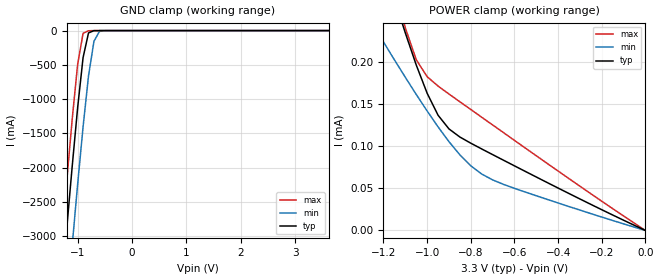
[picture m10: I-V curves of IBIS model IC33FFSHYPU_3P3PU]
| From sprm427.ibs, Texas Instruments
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|   Model IC33FFSHYPU_3P3PU
[Model]   IC33FFSHYPU_3P3PU
Model_type   Input
Polarity   Non-Inverting
Vinl =   0.9900V
Vinh =   2.3100V
C_comp   2.1548pF   2.1455pF   2.3140pF
[Temperature Range]   25.0000   0.1250k   -40.0000
[Voltage Range]   3.3000V   3.0000V   3.6000V
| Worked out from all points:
|   GND clamp passes 1 mA (typ) near -0.68 V on its own axis
|   POWER clamp passes 1 mA (typ) near -1.95 V on its own axis
[GND_clamp]
| voltage   I(typ)   I(min)   I(max)
-3.3V     -23.34A    -24.42A    -22.71A
-1.3V     -3.808A    -4.968A    -3.114A
-1.2V     -2.88A     -4.039A    -2.185A
-1.1V     -1.977A    -3.127A    -1.292A
-1V       -1.123A    -2.241A    -489.8mA
-900mV    -393.6mA   -1.402A    -39.47mA
-800mV    -34.19mA   -660.7mA   -2.615mA
-700mV    -1.201mA   -156.4mA   -443.3uA
-600mV    -178.7uA   -13.19mA   -224.2uA
-400mV    -135.4uA   -128.8uA   -210.3uA
3.62V     0A         0A         0A
[POWER_clamp]
| voltage   I(typ)   I(min)   I(max)
-3.3V     2.288mA    1.177mA    3.217mA
-1.25V    359.7uA    244.5uA    408.8uA
-1.2V     316.4uA    223.1uA    347.9uA
-1.1V     233.8uA    181.3uA    239.8uA
-1.05V    195.9uA    161uA      202.1uA
-1V       162.4uA    141.4uA    182uA
-950mV    136.4uA    122.6uA    170.9uA
-900mV    120.2uA    105.1uA    161.5uA
-800mV    103.3uA    76.55uA    143.2uA
-700mV    89.79uA    59.87uA    124.9uA
-450mV    56.72uA    36.8uA     79.36uA
0V        226.3pA    1.673nA    267.5pA
